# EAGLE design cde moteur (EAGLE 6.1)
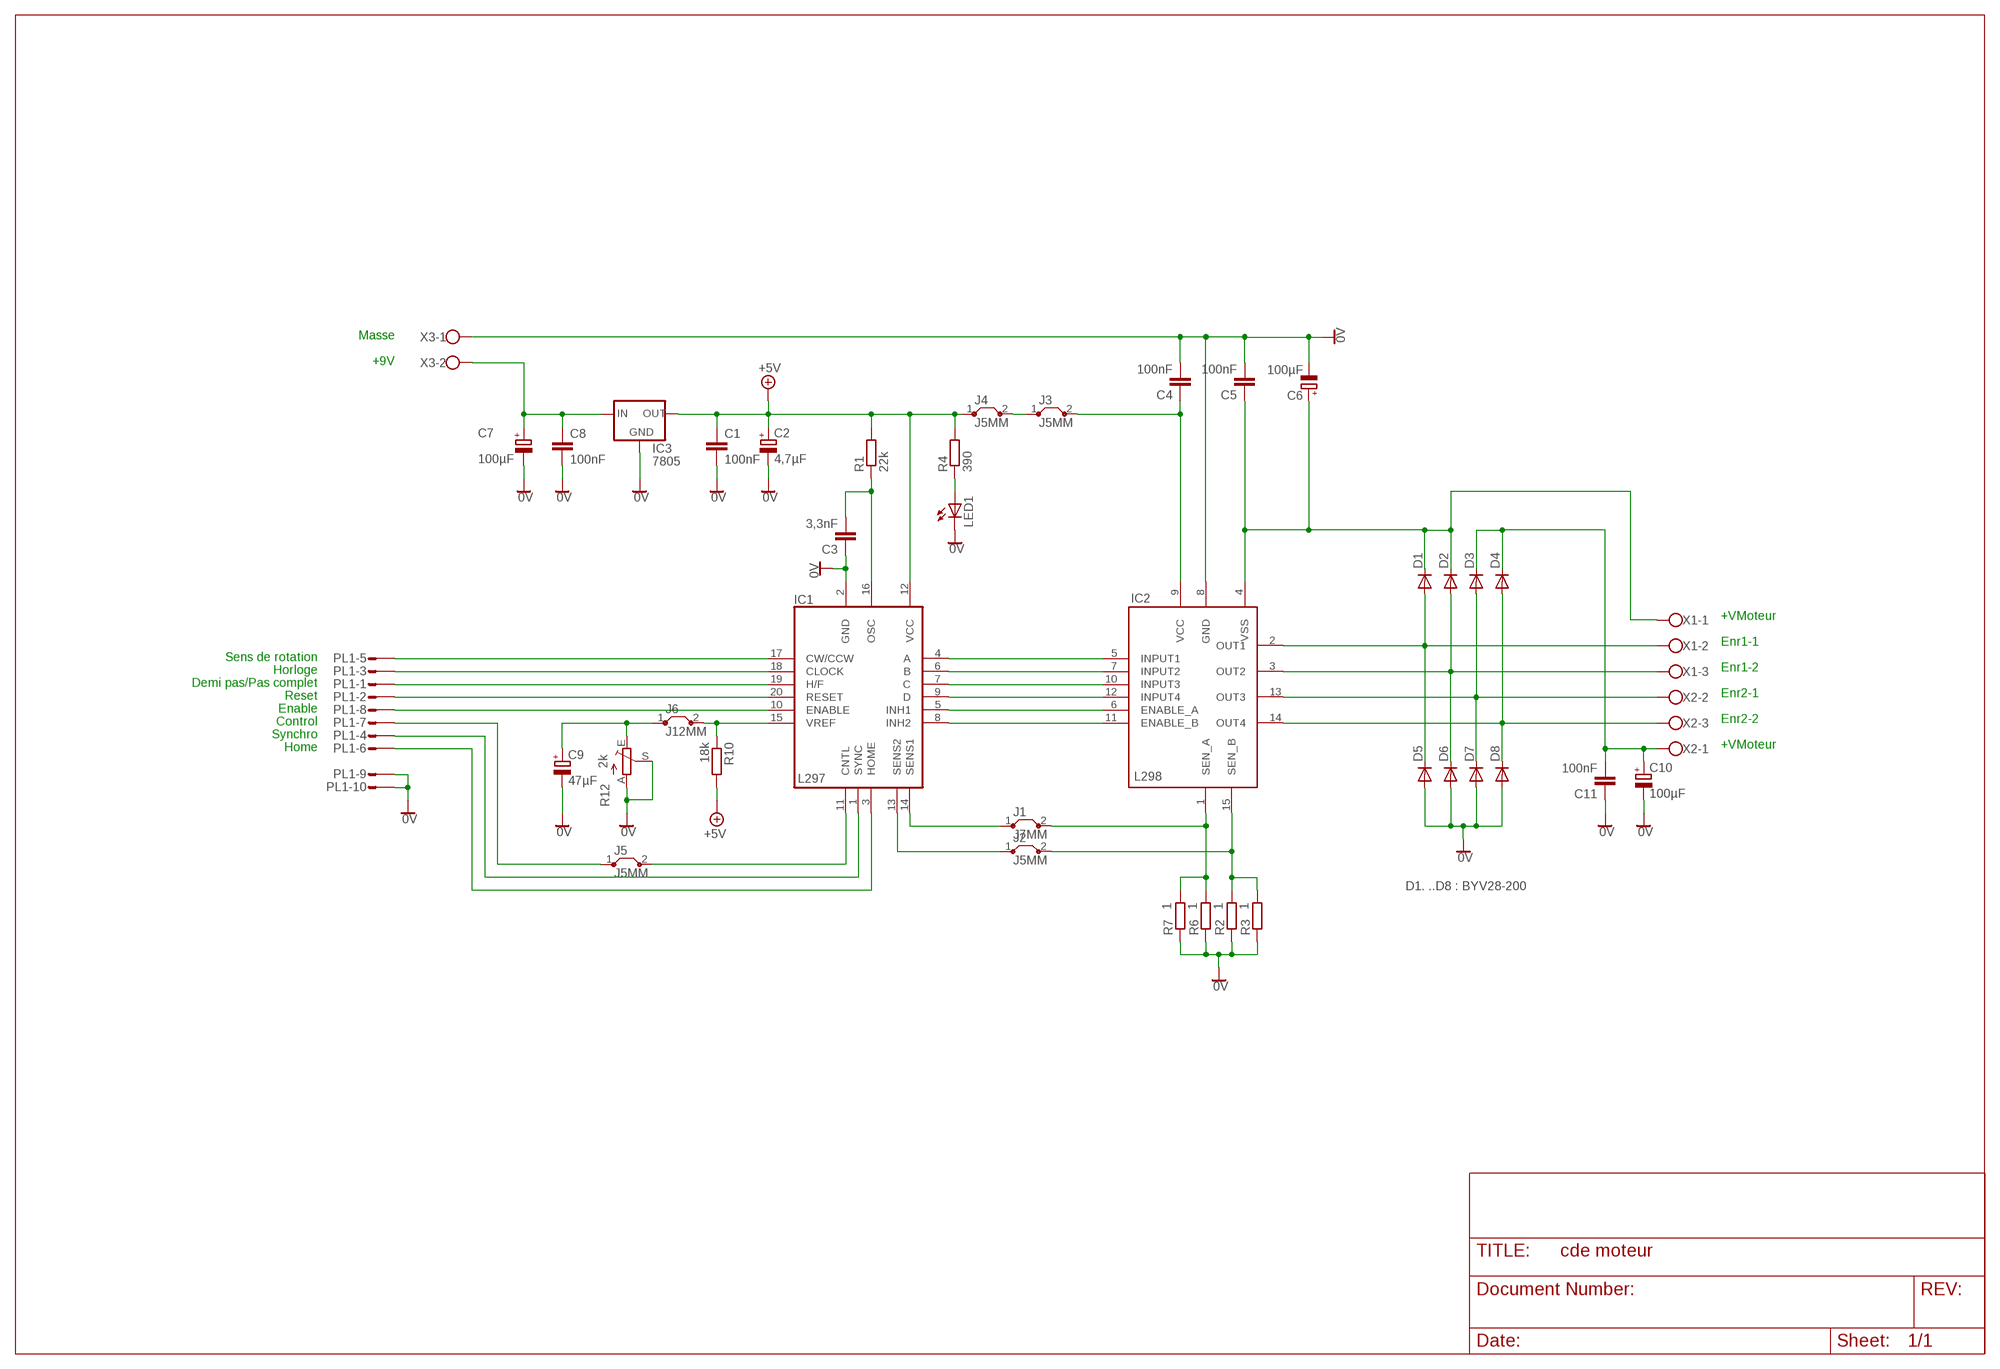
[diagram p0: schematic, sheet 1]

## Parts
C1  100nF  C-EU050-030X075  [C050-030X075]
C2  4,7µF  CPOL-EUE2.5-6  [E2,5-6]
C3  3,3nF  C-EU050-024X044  [C050-024X044]
C4  100nF  C-EU050-030X075  [C050-030X075]
C5  100nF  C-EU050-030X075  [C050-030X075]
C6  100µF  CPOL-EUE5-8.5  [E5-8,5]
C7  100µF  CPOL-EUE2.5-7  [E2,5-7]
C8  100nF  C-EU050-035X075  [C050-035X075]
C9  47µF  CPOL-EUE2.5-6  [E2,5-6]
C10  100µF  CPOL-EUE5-8.5  [E5-8,5]
C11  100nF  C-EU050-030X075  [C050-030X075]
D1  BYW55  [SOD57-10]
D2  BYW55  [SOD57-10]
D3  BYW55  [SOD57-10]
D4  BYW55  [SOD57-10]
D5  BYW55  [SOD57-10]
D6  BYW55  [SOD57-10]
D7  BYW55  [SOD57-10]
D8  BYW55  [SOD57-10]
IC1  L297  [DIL20]
IC2  L298  [MW-15]
IC3  7805  78XXS  [78XXS]
J1  J7MM  [07]
J2  J5MM  [05]
J3  J5MM  [05]
J4  J5MM  [05]
J5  J5MM  [05]
J6  J12MM  [12]
LED1  LED3MM  [LED3MM]
PL1  10HS  [10H]
R1  22k  R-EU_0207/10  [0207/10]
R2  1  R-EU_0309/12  [0309/12]
R3  1  R-EU_0309/12  [0309/12]
R4  390  R-EU_0207/10  [0207/10]
R6  1  R-EU_0309/12  [0309/12]
R7  1  R-EU_0309/12  [0309/12]
R10  18k  R-EU_0207/10  [0207/10]
R12  2k  TRIM_EU-PTSPIN  [PT-SPIN]
X1  W237-103  [W237-103]
X2  W237-103  [W237-103]
X3  W237-102  [W237-102]

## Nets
0V: C1.2 C2.- C3.1 C4.2 C5.2 C6.- C7.- C8.2 C9.- C10.- C11.1 D5.A D6.A D7.A D8.A IC1.2(GND) IC2.8(GND) IC3.GND LED1.K(C) PL1.9 PL1.10 R2.1 R3.1 R6.1 R7.1 R12.A R12.S X3.1
+5V: C1.1 C2.+ IC1.12(VCC) IC3.OUT J4.1 R1.2 R4.2 R10.2
N$1: IC1.4(A) IC2.5(INPUT1)
N$2: IC1.6(B) IC2.7(INPUT2)
N$3: IC1.7(C) IC2.10(INPUT3)
N$4: IC1.9(D) IC2.12(INPUT4)
N$5: IC1.5(INH1) IC2.6(ENABLE_A)
N$6: IC1.8(INH2) IC2.11(ENABLE_B)
N$7: D1.A D5.C IC2.2(OUT1) X1.2
N$8: C3.2 IC1.16(OSC) R1.1
N$9: D2.A D6.C IC2.3(OUT2) X1.3
N$10: D3.A D7.C IC2.13(OUT3) X2.2
N$11: D4.A D8.C IC2.14(OUT4) X2.3
N$12: IC2.1(SEN_A) J1.2 R6.2 R7.2
N$13: C5.1 C6.+ D1.C D2.C IC2.4(VSS) X1.1
N$14: IC2.15(SEN_B) J2.2 R2.2 R3.2
N$15: C7.+ C8.1 IC3.IN X3.2
N$17: C10.+ C11.2 D3.C D4.C X2.1
N$19: IC1.20(RESET) PL1.2
N$20: IC1.19(H/F) PL1.1
N$21: IC1.18(CLOCK) PL1.3
N$22: IC1.17(CW/CCW) PL1.5
N$23: IC1.10(ENABLE) PL1.8
N$24: J5.1 PL1.7
N$25: IC1.1(SYNC) PL1.4
N$26: IC1.3(HOME) PL1.6
N$27: C9.+ J6.1 R12.E
N$29: IC1.14(SENS1) J1.1
N$30: IC1.13(SENS2) J2.1
N$31: C4.1 IC2.9(VCC) J3.2
N$32: J3.1 J4.2
N$33: IC1.11(CNTL) J5.2
N$34: IC1.15(VREF) J6.2 R10.1
N$101: LED1.A R4.1

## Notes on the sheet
- Masse
- +9V
- +VMoteur
- Enr1-1
- Sens de rotation
- Horloge
- Enr1-2
- Demi pas/Pas complet
- Reset
- Enr2-1
- Enable
- Control
- Enr2-2
- Synchro
- Home
- +VMoteur
- D1. ..D8 : BYV28-200

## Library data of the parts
C1 C3-C5 C8 C11 = rcl:C-EU: CAPACITOR, European symbol
C2 C6 C7 C9 C10 = rcl:CPOL-EU: POLARIZED CAPACITOR, European symbol
D1-D8 = diode:BYW55: DIODE
IC1 = sgs-thom:L297
IC2 = sgs-thom:L298
IC3 = v-reg:78XXS: VOLTAGE REGULATOR
J1-J6 = jumper:J: Bridge
LED1 = led:LED: LED
PL1 = con-harting-h:10HS: CONNECTOR
R1-R4 R6 R7 R10 = rcl:R-EU_: RESISTOR, European symbol
R12 = pot:TRIM_EU-: POTENTIOMETER
X1 X2 = con-wago-500:W237-103: WAGO SCREW CLAMP
X3 = con-wago-500:W237-102: WAGO SCREW CLAMP

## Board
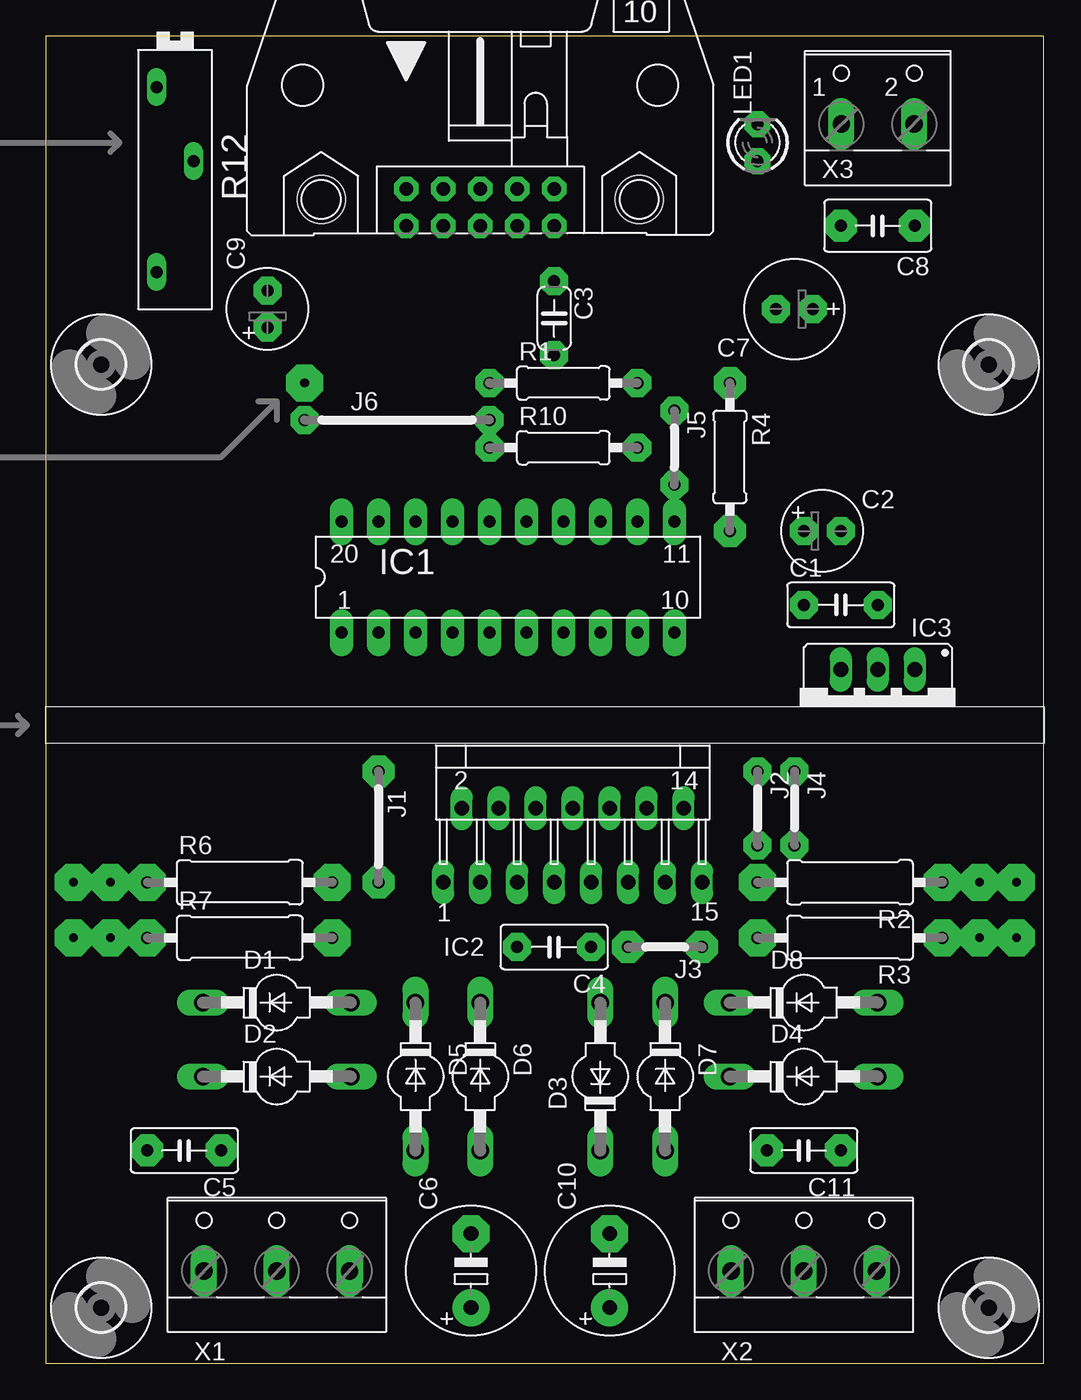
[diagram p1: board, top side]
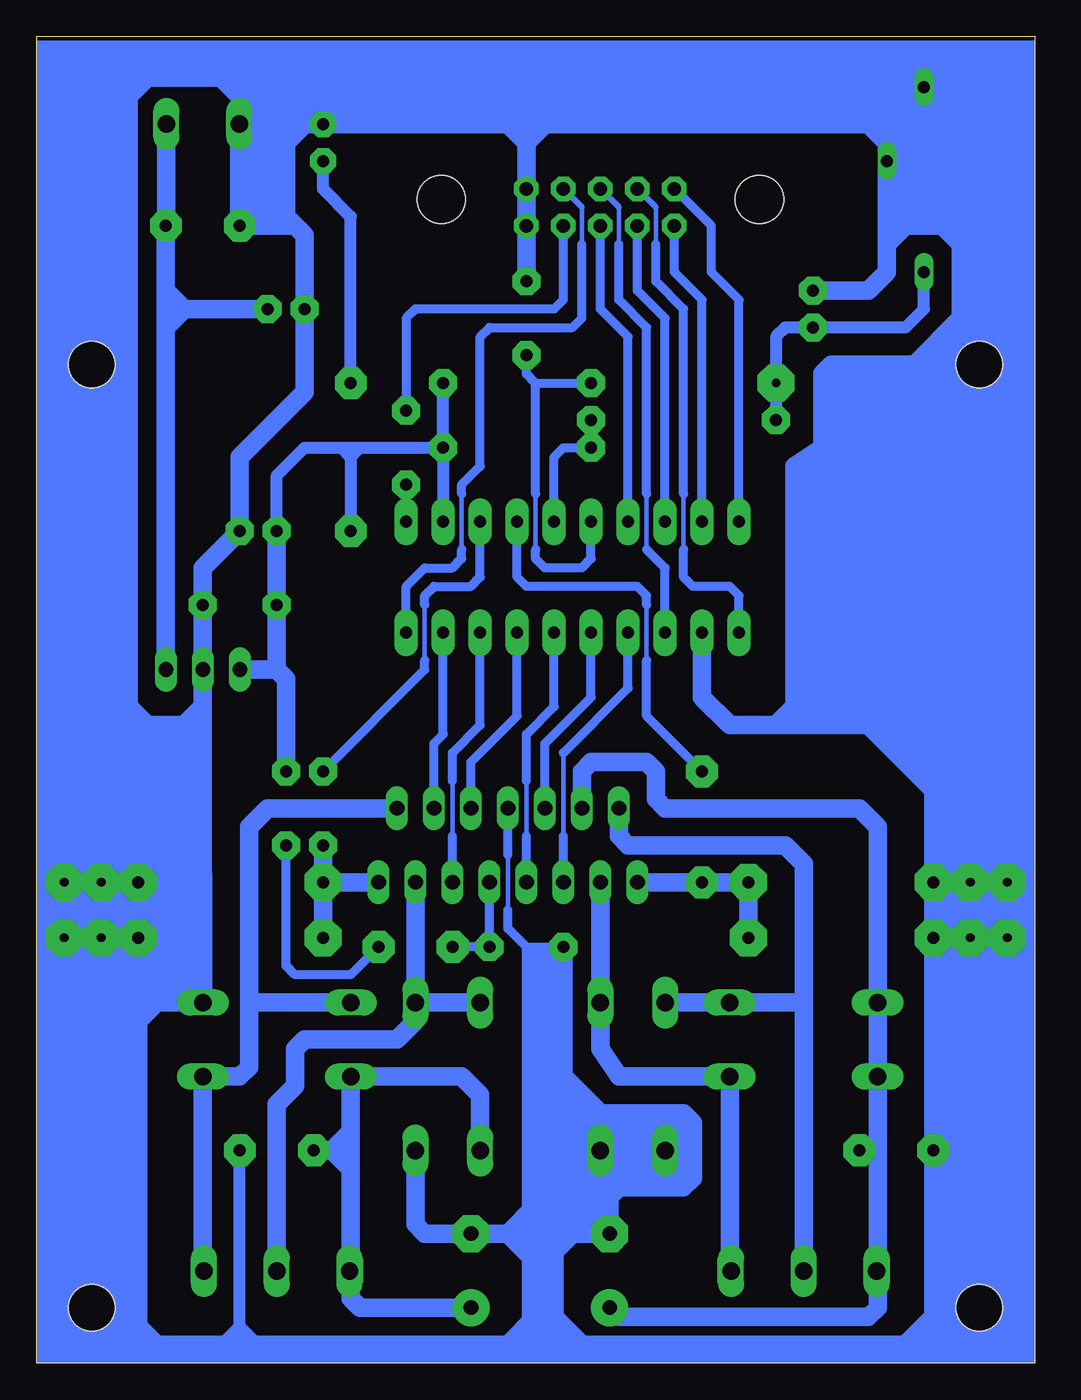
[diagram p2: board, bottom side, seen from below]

Size 68.56 x 91.11 mm. Coordinates in mm from the lower left corner, seen from the top.
Outline: 0,0 68.56,0 68.56,91.11 0,91.11 0,0
Copper layers (1*16): Top 0.035mm / dielectric 1.5mm / Bottom 0.035mm
Design rules: minimum track width 10mil, minimum drill 24mil, track to track 8mil, track to pad 8mil, pad to pad 8mil, via to via 8mil, smd to smd 8mil, copper to edge 40mil, drill to drill 8mil, minimum pad ring 10mil, minimum via ring 8mil, stop-mask expansion 4mil, vias tented up to drill 0mil, thermal gap 10mil

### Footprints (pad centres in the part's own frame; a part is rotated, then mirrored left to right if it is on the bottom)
C050-030X075 = drill 0.813 octagon: 1 -2.54,0; 2 2.54,0
E2,5-6 = drill 0.813 pad 1.6: + -1.27,0 | drill 0.813 pad 1.6 octagon: - 1.27,0
C050-024X044 = drill 0.813 octagon: 1 -2.54,0; 2 2.54,0
E5-8,5 = drill 1.016 pad 2.54: + -2.54,0 | drill 1.016 pad 2.54 octagon: - 2.54,0
E2,5-7 = drill 0.813 pad 1.6: + -1.27,0 | drill 0.813 pad 1.6 octagon: - 1.27,0
C050-035X075 = drill 0.813 octagon: 1 -2.54,0; 2 2.54,0
SOD57-10 = drill 1.194 long: A 5.08,0; C -5.08,0
DIL20 = drill 0.813 pad 1.6 long: 1 -11.43,-3.81; 2 -8.89,-3.81; 3 -6.35,-3.81; 4 -3.81,-3.81; 5 -1.27,-3.81; 6 1.27,-3.81; 7 3.81,-3.81; 8 6.35,-3.81; 9 8.89,-3.81; 10 11.43,-3.81; 11 11.43,3.81; 12 8.89,3.81; 13 6.35,3.81; 14 3.81,3.81; 15 1.27,3.81; 16 -1.27,3.81; 17 -3.81,3.81; 18 -6.35,3.81; 19 -8.89,3.81; 20 -11.43,3.81
MW-15 = drill 1.016 pad 1.27 long: 1 -8.89,-5.08; 2 -7.62,0; 3 -6.35,-5.08; 4 -5.08,0; 5 -3.81,-5.08; 6 -2.54,0; 7 -1.27,-5.08; 8 0,0; 9 1.27,-5.08; 10 2.54,0; 11 3.81,-5.08; 12 5.08,0; 13 6.35,-5.08; 14 7.62,0; 15 8.89,-5.08
78XXS = drill 1.016 long: GND 0,-2.54; IN -2.54,-2.54; OUT 2.54,-2.54
07 = drill 0.813 pad 1.6 octagon: 1 -3.81,0; 2 3.81,0
05 = drill 0.813 pad 1.6 octagon: 1 -2.54,0; 2 2.54,0
12 = drill 0.813 pad 1.6 octagon: 1 -6.35,0; 2 6.35,0
LED3MM = drill 0.813 octagon: A -1.27,0; K 1.27,0
10H = drill 0.914: 1 -5.08,-1.27 | drill 0.914 octagon: 2 -5.08,1.27; 3 -2.54,-1.27; 4 -2.54,1.27; 5 0,-1.27; 6 0,1.27; 7 2.54,-1.27; 8 2.54,1.27; 9 5.08,-1.27; 10 5.08,1.27 | hole 3.302: -10.922,0.533; 10.922,0.533
0207/10 = drill 0.813 octagon: 1 -5.08,0; 2 5.08,0
0309/12 = drill 0.813 octagon: 1 -6.35,0; 2 6.35,0
PT-SPIN = drill 0.813 long: A -6.35,-1.27; E 6.35,-1.27; S -1.27,1.27
3,2 = hole 3.2: 0,0
W237-103 = drill 1.194 long: 1 -5,-1.29; 2 0,-1.29; 3 5,-1.29
W237-102 = drill 1.194 long: 1 -2.5,-1.27; 2 2.5,-1.27

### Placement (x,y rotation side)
C1  54.61,52.07 0 top
C2  53.34,57.15 0 top
C3  34.92,71.76 270 top
C4  34.92,28.57 180 top
C5  9.52,14.61 180 top
C6  29.21,6.35 90 top
C7  51.44,72.39 180 top
C8  57.15,78.11 180 top
C9  15.24,72.39 90 top
C10  38.73,6.35 90 top
C11  52.07,14.61 180 top
D1  15.88,24.77 0 top
D2  15.88,19.68 0 top
D3  38.1,19.68 90 top
D4  52.07,19.68 0 top
D5  25.4,19.68 270 top
D6  29.84,19.68 270 top
D7  42.55,19.68 270 top
D8  52.07,24.77 0 top
IC1  31.75,53.97 0 top
IC2  36.2,38.1 0 top
IC3  57.15,45.08 180 top
J1  22.86,36.83 270 top
J2  48.9,38.1 270 top
J3  42.55,28.57 180 top
J4  51.44,38.1 270 top
J5  43.18,62.87 270 top
J6  24.13,64.77 0 top
LED1  48.9,83.82 90 top
PL1  29.84,79.38 0 top
R1  35.56,67.31 0 top
R2  55.25,33.02 180 top
R3  55.25,29.21 180 top
R4  46.99,62.23 270 top
R6  13.34,33.02 0 top
R7  13.34,29.21 0 top
R10  35.56,62.87 0 top
R12  8.89,81.28 270 top
U$1  [3,2]  3.81,3.81 0 top
U$2  [3,2]  64.77,3.81 0 top
U$3  [3,2]  3.81,68.58 0 top
U$4  [3,2]  64.77,68.58 0 top
X1  15.88,7.62 0 top
X2  52.07,7.62 0 top
X3  57.15,86.36 0 top

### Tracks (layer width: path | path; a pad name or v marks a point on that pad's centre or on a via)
0V
  Bottom 0.305: 36.2,31.11 36.2,34.92
  Bottom 0.406: 10.16,85.09 10.16,85.73 | C8.2 54.65,78.15
  Bottom 0.61: D5.A D6.A 34.92,14.61 | 34.92,28.57 36.2,29.84 36.2,31.11 | 36.2,34.92 IC2.8 | 34.92,14.61 34.92,8.89 34.92,1.27 | 34.92,14.61 34.92,28.57 | 34.92,28.57 C4.2
  Bottom 0.813: 54.61,1.27 54.61,2.54 | 54.61,2.54 C11.1 | 54.61,2.54 55.88,1.27 | 53.34,1.27 54.61,2.54
  Bottom 1.27: 6.98,3.18 6.98,1.9 7.62,1.27 8.89,1.27 | 6.98,3.18 C5.2 6.98,28.57 7.62,29.21 R7.1 R6.1 6.98,39.37 11.43,43.81 16.51,43.81 | 8.89,1.27 31.12,1.27 | 31.12,1.27 34.92,1.27 36.2,1.27 | 36.2,1.27 53.34,1.27 54.61,1.27 55.88,1.27 60.33,1.27 61.59,2.54 61.59,23.5 | 61.59,23.5 61.59,24.77 | 61.59,24.77 61.59,26.04 | 61.59,26.04 R3.1 R2.1 57.79,33.02 57.15,33.65 57.15,45.08 | 61.59,24.77 60.33,24.77 | 60.33,24.77 D8.A | 36.2,8.89 34.92,8.89 31.75,8.89 | 36.2,8.89 C10.- 41.91,8.89 42.55,9.53 D7.A | 31.75,8.89 C6.- | 57.15,45.08 IC3.GND C1.2 57.15,54.61 C2.- 54.61,62.23 50.16,66.67 C7.- 50.16,77.47 50.8,78.11 | 50.8,78.11 51.44,78.11 | 51.44,78.11 C8.2 | 10.16,83.82 R12.S 10.16,78.11 | 10.16,83.82 10.16,85.73 10.16,87 9.52,87.63 R12.A | 11.43,85.09 10.16,85.09 | 33.66,85.09 11.43,85.09 | 34.92,84.45 33.66,85.09 | 34.92,84.45 34.92,83.82 | 34.92,83.82 PL1.10 PL1.9 C3.1 | 16.51,43.81 17.78,43.81 | 17.78,43.81 20.95,43.81 22.86,45.72 IC1.2 | 10.16,76.84 10.16,74.93 11.43,73.66 C9.- | 10.16,78.11 10.16,76.84 | 36.2,85.09 34.92,84.45 | 50.16,85.09 X3.1 54.65,78.15 | 50.16,85.09 LED1.K 36.2,85.09 | 16.51,43.81 16.51,45.08 | 16.51,45.08 16.51,61.59 14.61,62.87 14.61,67.95 13.97,68.58 8.25,68.58 5.08,71.76 5.08,89.54 0.63,89.54 0.63,44.45 | 10.16,78.11 8.89,78.11 | 8.89,78.11 6.35,78.11 | 6.35,78.11 5.71,78.11 4.44,76.84 | 34.92,83.82 33.66,85.09 | 36.2,85.09 34.92,83.82 | 10.16,76.84 8.89,78.11 | 6.35,78.11 4.44,76.2 | 11.43,85.09 10.16,83.82 | 54.61,87 54.61,85.73 | 54.61,87 54.61,87.63 55.25,88.27 55.88,88.27 | 55.88,88.27 60.96,88.27 62.23,87 62.23,45.08 60.96,43.81 58.42,43.81 57.15,45.08 | 61.59,23.5 60.33,24.77 | 60.33,24.77 61.59,26.04
  Bottom 1.27: 36.2,8.89 34.29,10.79 | 36.2,8.89 34.29,6.99 | 36.2,1.27 34.29,3.18 | 33.66,3.18 33.02,3.18 31.12,1.27 | 31.75,8.89 33.02,7.62 | 17.78,43.81 16.51,45.08 | 55.88,88.27 54.61,87 | 6.98,3.18 8.89,1.27 | 51.44,78.11 51.44,83.82 50.16,85.09 | 50.8,78.11 52.07,79.38
+5V
  Bottom 0.813: R10.2 R1.2 | R10.2 IC1.12 | C2.+ 52.07,60.96 50.16,62.87 47.62,62.87 | 47.62,62.87 46.99,62.87 | 46.99,62.87 46.36,62.87 | 46.36,62.87 R10.2 | 46.99,62.87 46.99,62.23 | 46.99,62.23 R4.2 | 46.99,62.23 46.36,62.87 | 46.99,62.23 47.62,62.87
  Bottom 1.27: C2.+ C1.1 52.07,47.62 | 52.07,47.62 IC3.OUT | J4.1 51.44,46.99 52.07,47.62
N$1
  Bottom 0.305: 32.38,36.2 32.38,40 32.38,41.91
  Bottom 0.61: IC1.4 27.94,46.35 32.38,41.91 | IC2.5 32.38,36.2
N$2
  Bottom 0.305: 34.92,36.2 34.92,40
  Bottom 0.61: IC1.6 33.02,45.08 34.92,43.18 34.92,40 | IC2.7 34.92,36.2
N$3
  Bottom 0.61: IC1.7 35.56,44.45 38.73,41.27 IC2.10
N$4
  Bottom 0.61: IC1.9 40.64,43.18 41.27,42.54 IC2.12
N$5
  Bottom 0.61: IC1.5 30.48,45.72 33.66,42.54 IC2.6
N$6
  Bottom 0.305: 40.01,36.2 40.01,40
  Bottom 0.61: IC1.8 38.1,43.81 40.01,41.91 40.01,40 | IC2.11 40.01,36.2
N$7
  Bottom 1.27: D5.C D1.A 15.88,24.77 | X1.2 15.88,24.77 | 15.88,24.77 15.88,34.29 17.14,35.56 27.94,35.56 28.58,36.2 IC2.2
N$8
  Bottom 0.305: 34.29,55.88 34.29,59.69
  Bottom 0.61: 34.29,67.31 R1.1 | 34.29,67.31 34.92,67.95 C3.2 | IC1.16 30.48,55.24 31.12,54.61 33.66,54.61 34.29,55.24 34.29,55.88 | 34.29,59.69 34.29,67.31
N$9
  Bottom 0.406: X1.3 20.95,6.41
  Bottom 1.27: IC2.3 D6.C 29.84,21.59 28.58,19.68 D2.A 20.95,6.41
N$10
  Bottom 1.27: D7.C IC2.13 | D7.C D3.A | D7.C 42.55,23.5 43.82,22.23 50.16,22.23 50.8,21.59 50.8,19.05 52.07,17.78 X2.2
N$11
  Bottom 0.406: X2.3 57.15,6.41
  Bottom 1.27: 53.98,24.77 D8.C | 53.98,24.77 53.98,20.32 54.61,19.68 D4.A 57.15,6.41 | IC2.14 52.7,38.1 53.98,36.83 53.98,24.77
N$12
  Bottom 1.27: R7.2 R6.2 | R6.2 J1.2 | R6.2 IC2.1
N$13
  Bottom 0.406: 10.79,6.41 X1.1 10.79,6.25
  Bottom 0.61: 10.79,14.61 C5.1
  Bottom 1.27: IC2.4 31.12,40.64 30.48,41.27 26.67,41.27 26.03,40.64 26.03,38.73 25.4,38.1 12.06,38.1 10.79,36.83 D1.C D2.C 10.79,14.61 10.79,6.41 | C6.+ 28.58,3.18 11.43,3.18 10.79,3.81 10.79,6.25
N$14
  Bottom 1.27: R2.2 IC2.15 | R3.2 R2.2 | R2.2 J2.2
N$15
  Bottom 0.406: 59.61,78.19 C8.1 59.65,78.15
  Bottom 1.27: 59.69,72.39 59.69,73.66 | 59.69,73.66 C8.1 | 59.69,72.39 58.42,72.39 | 58.42,72.39 C7.+ | 59.65,78.15 X3.2 | IC3.IN 59.69,71.12 | 59.69,71.12 59.69,72.39 | 58.42,72.39 59.69,73.66 | 59.69,71.12 58.42,72.39
N$16  (via drill 0.6 pad 2.54)
  other vias: 4.44,33.02
N$17
  Bottom 0.406: 46.99,6.41 X2.1 46.99,6.25
  Bottom 1.27: D3.C 38.1,18.41 39.37,19.68 D4.C 46.99,15.88 | 46.99,6.41 46.99,13.34 | 46.99,13.34 46.99,14.61 | 46.99,14.61 46.99,15.88 | C10.+ 46.36,3.81 46.99,4.45 46.99,6.25 | 46.99,14.61 48.26,14.61 | 48.26,14.61 C11.2 | 48.26,14.61 46.99,15.88 | 46.99,13.34 48.26,14.61
N$19
  Bottom 0.61: IC1.20 20.32,73.03 22.23,74.93 22.23,78.11 PL1.2
N$20
  Bottom 0.61: IC1.19 22.86,73.03 24.77,74.93 PL1.1
N$21
  Bottom 0.61: IC1.18 25.4,71.76 27.3,73.66 PL1.3
N$22
  Bottom 0.61: IC1.17 27.94,70.48 29.84,72.39 PL1.5
N$23
  Bottom 0.305: 39.37,55.88 39.37,59.69 | 31.12,76.84 31.12,79.38
  Bottom 0.406: 31.12,79.38 PL1.8
  Bottom 0.61: IC1.10 43.18,53.34 41.91,54.61 40.01,54.61 39.37,55.24 39.37,55.88 | 39.37,59.69 39.37,60.32 38.1,61.59 38.1,70.48 37.46,71.12 31.75,71.12 31.12,71.76 31.12,76.84
N$24
  Bottom 0.61: PL1.7 32.38,73.03 33.02,72.39 42.55,72.39 43.18,71.76 J5.1
N$25
  Bottom 0.305: 24.13,55.88 24.13,59.69 | 26.03,76.84 26.03,79.38
  Bottom 0.406: 26.03,79.38 PL1.4
  Bottom 0.61: IC1.1 20.32,52.7 20.95,53.34 23.49,53.34 24.13,53.97 24.13,55.88 | 24.13,59.69 24.13,72.39 26.03,74.3 26.03,76.84
N$26
  Bottom 0.305: 26.67,55.88 26.67,59.69 | 28.58,76.84 28.58,79.38
  Bottom 0.406: 28.58,79.38 PL1.6
  Bottom 0.61: IC1.3 25.4,54.61 26.67,55.88 | 26.67,59.69 26.67,71.12 28.58,73.03 28.58,76.84
N$27  (via drill 0.6 pad 2.54)
  Bottom 0.813: R12.E 7.62,72.39 8.89,71.12 C9.+ 17.14,71.12 17.78,70.48 v17.78,67.31 J6.1
N$29
  Bottom 0.305: 26.67,48.26 26.67,52.07
  Bottom 0.61: J1.1 26.67,44.45 26.67,48.26 | 26.67,52.07 26.67,52.7 27.3,53.34 34.92,53.34 35.56,53.97 IC1.14
N$30
  Bottom 0.305: 41.91,48.26 41.91,52.07
  Bottom 0.61: J2.1 41.91,47.62 41.91,48.26 | 41.91,52.07 41.91,52.7 41.27,53.34 38.73,53.34 38.1,53.97 IC1.13
N$31
  Bottom 0.61: IC2.9 C4.1 J3.2
N$32
  Bottom 0.61: J3.1 46.99,26.67 50.8,26.67 51.44,27.3 J4.2
N$33
  Bottom 0.406: IC1.11 J5.2
N$34
  Bottom 0.61: IC1.15 33.02,62.23 32.38,62.87 R10.1 J6.2
N$35  (via drill 0.6 pad 2.54)
  other vias: 3.81,68.58
N$36  (via drill 0.6 pad 2.54)
  other vias: 64.77,68.58
N$37  (via drill 0.6 pad 2.54)
  other vias: 18.97,79.92
N$38  (via drill 0.6 pad 2.54)
  other vias: 40.78,79.92
N$39  (via drill 0.6 pad 1.68)
  other vias: 24.77,78.11
N$40  (via drill 0.6 pad 1.68)
  other vias: 24.77,80.65
N$41  (via drill 0.6 pad 1.68)
  other vias: 29.84,78.11
N$42  (via drill 0.6 pad 1.68)
  other vias: 27.3,78.11
N$43  (via drill 0.6 pad 1.68)
  other vias: 27.3,80.65
N$44  (via drill 0.6 pad 1.68)
  other vias: 29.84,80.65
N$45  (via drill 0.6 pad 1.68)
  other vias: 32.38,78.11
N$46  (via drill 0.6 pad 1.68)
  other vias: 32.38,80.65
N$47  (via drill 0.6 pad 1.68)
  other vias: 34.92,78.11
N$48  (via drill 0.6 pad 1.68)
  other vias: 34.92,80.65
N$49  (via drill 0.6 pad 2.54)
  other vias: 3.81,3.81
N$50  (via drill 0.6 pad 2.54)
  other vias: 64.77,3.81
N$51  (via drill 0.6 pad 2.18)
  other vias: 49.53,14.61
N$52  (via drill 0.6 pad 2.18)
  other vias: 54.61,14.61
N$53  (via drill 0.6 pad 2.18)
  other vias: 12.06,14.61
N$54  (via drill 0.6 pad 2.18)
  other vias: 6.98,14.61
N$55  (via drill 0.6 pad 2.18)
  other vias: 45.09,28.57
N$56  (via drill 0.6 pad 2.18)
  other vias: 40.01,28.57
N$57  (via drill 0.6 pad 1.93)
  other vias: 37.46,28.57
N$58  (via drill 0.6 pad 1.68, 0.6 pad 1.93)
  Bottom 1.27: v32.38,28.57 32.38,19.68 29.84,17.14 24.13,17.14 23.49,16.51 23.49,12.7 24.13,12.07 28.58,12.07 29.21,11.43 v29.21,8.89
N$59  (via drill 0.6 pad 2.54)
  other vias: 48.9,33.02
N$60  (via drill 0.6 pad 2.54)
  other vias: 61.59,33.02
N$61  (via drill 0.6 pad 2.54)
  other vias: 48.9,29.21
N$62  (via drill 0.6 pad 2.54)
  other vias: 61.59,29.21
N$63  (via drill 0.6 pad 1.93)
  other vias: 48.9,35.56
N$64  (via drill 0.6 pad 1.93)
  other vias: 51.44,35.56
N$65  (via drill 0.6 pad 1.93)
  other vias: 48.9,40.64
N$66  (via drill 0.6 pad 1.93)
  other vias: 51.44,40.64
N$67  (via drill 0.6 pad 1.93)
  other vias: 57.15,52.07
N$68  (via drill 0.6 pad 1.93)
  other vias: 52.07,52.07
N$69  (via drill 0.6 pad 2.18)
  other vias: 22.86,40.64
N$70  (via drill 0.6 pad 2.18)
  other vias: 22.86,33.02
N$71  (via drill 0.6 pad 2.54)
  other vias: 19.69,33.02
N$72  (via drill 0.6 pad 2.54)
  other vias: 19.69,29.21
N$73  (via drill 0.6 pad 2.54)
  other vias: 6.98,33.02
N$74  (via drill 0.6 pad 2.54)
  other vias: 6.98,29.21
N$75  (via drill 0.6 pad 1.93)
  other vias: 30.48,62.87
N$76  (via drill 0.6 pad 1.93)
  other vias: 30.48,64.77
N$77  (via drill 0.6 pad 1.93)
  other vias: 30.48,67.31
N$78  (via drill 0.6 pad 1.93)
  other vias: 17.78,64.77
N$79  (via drill 0.6 pad 1.68)
  other vias: 10.79,6.35
N$80  (via drill 0.6 pad 1.68)
  other vias: 15.88,6.35
N$81  (via drill 0.6 pad 1.68)
  other vias: 20.95,6.35
N$82  (via drill 0.6 pad 1.68)
  other vias: 46.99,6.35
N$83  (via drill 0.6 pad 1.68)
  other vias: 52.07,6.35
N$84  (via drill 0.6 pad 1.68)
  other vias: 57.15,6.35
N$85  (via drill 0.6 pad 1.68)
  other vias: 10.79,19.68
N$86  (via drill 0.6 pad 1.68)
  other vias: 10.79,24.77
N$87  (via drill 0.6 pad 1.68)
  other vias: 20.95,24.77
N$88  (via drill 0.6 pad 1.68)
  other vias: 20.95,19.68
N$89  (via drill 0.6 pad 1.68)
  other vias: 25.4,24.77
N$90  (via drill 0.6 pad 1.68)
  other vias: 29.84,24.77
N$91  (via drill 0.6 pad 1.68)
  other vias: 25.4,14.61
N$92  (via drill 0.6 pad 1.68)
  other vias: 29.84,14.61
N$93  (via drill 0.6 pad 1.68)
  other vias: 46.99,24.77
N$94  (via drill 0.6 pad 1.68)
  other vias: 57.15,24.77
N$95  (via drill 0.6 pad 1.68)
  other vias: 57.15,19.68
N$96  (via drill 0.6 pad 1.68)
  other vias: 46.99,19.68
N$97  (via drill 0.6 pad 1.68)
  other vias: 38.1,24.77
N$98  (via drill 0.6 pad 1.68)
  other vias: 42.55,24.77
N$99  (via drill 0.6 pad 1.68)
  other vias: 42.55,14.61
N$100  (via drill 0.6 pad 1.68)
  other vias: 38.1,14.61
N$101
  Bottom 0.813: R4.1 46.99,78.74 48.9,80.65 LED1.A
N$102  (via drill 0.6 pad 1.68)
  other vias: 29.21,3.81
N$103  (via drill 0.6 pad 1.68)
  other vias: 38.73,3.81
N$104  (via drill 0.6 pad 1.68)
  other vias: 38.73,8.89
N$105  (via drill 0.6 pad 1.27)
  other vias: 28.58,38.1
N$106  (via drill 0.6 pad 1.27)
  other vias: 43.82,38.1
N$107  (via drill 0.6 pad 1.27)
  other vias: 41.27,38.1
N$108  (via drill 0.6 pad 1.27)
  other vias: 38.73,38.1
N$109  (via drill 0.6 pad 1.27)
  other vias: 36.2,38.1
N$110  (via drill 0.6 pad 1.27)
  other vias: 33.66,38.1
N$111  (via drill 0.6 pad 1.27)
  other vias: 31.12,38.1
N$112  (via drill 0.6 pad 1.27)
  other vias: 45.09,33.02
N$113  (via drill 0.6 pad 1.27)
  other vias: 42.55,33.02
N$114  (via drill 0.6 pad 1.27)
  other vias: 40.01,33.02
N$115  (via drill 0.6 pad 1.27)
  other vias: 37.46,33.02
N$116  (via drill 0.6 pad 1.27)
  other vias: 32.38,33.02
N$117  (via drill 0.6 pad 1.27)
  other vias: 34.92,33.02
N$118  (via drill 0.6 pad 1.27)
  other vias: 29.84,33.02
N$119  (via drill 0.6 pad 1.27)
  other vias: 27.3,33.02
N$120  (via drill 0.6 pad 1.27)
  other vias: 54.61,47.62
N$121  (via drill 0.6 pad 1.27)
  other vias: 57.15,47.62
N$122  (via drill 0.6 pad 1.27)
  other vias: 59.69,47.62
N$123  (via drill 0.6 pad 1.27)
  other vias: 20.32,57.78
N$124  (via drill 0.6 pad 1.27)
  other vias: 20.32,50.16
N$125  (via drill 0.6 pad 1.27)
  other vias: 22.86,50.16
N$126  (via drill 0.6 pad 1.27)
  other vias: 25.4,50.16
N$127  (via drill 0.6 pad 1.27)
  other vias: 38.1,57.78
N$128  (via drill 0.6 pad 1.27)
  other vias: 33.02,57.78
N$129  (via drill 0.6 pad 1.27)
  other vias: 27.94,57.78
N$130  (via drill 0.6 pad 1.27)
  other vias: 25.4,57.78
N$131  (via drill 0.6 pad 1.27)
  other vias: 22.86,57.78
N$132  (via drill 0.6 pad 1.27)
  other vias: 30.48,57.78
N$133  (via drill 0.6 pad 1.27)
  other vias: 35.56,57.78
N$134  (via drill 0.6 pad 1.27)
  other vias: 40.64,57.78
N$135  (via drill 0.6 pad 1.27)
  other vias: 43.18,57.78
N$136  (via drill 0.6 pad 1.27)
  other vias: 33.02,50.16
N$137  (via drill 0.6 pad 1.27)
  other vias: 30.48,50.16
N$138  (via drill 0.6 pad 1.27)
  other vias: 27.94,50.16
N$139  (via drill 0.6 pad 1.27)
  other vias: 35.56,50.16
N$140  (via drill 0.6 pad 1.27)
  other vias: 38.1,50.16
N$141  (via drill 0.6 pad 1.27)
  other vias: 40.64,50.16
N$142  (via drill 0.6 pad 1.27)
  other vias: 43.18,50.16
N$143  (via drill 0.6 pad 1.93)
  other vias: 43.18,60.32
N$144  (via drill 0.6 pad 1.93)
  other vias: 43.18,65.41
N$145  (via drill 0.6 pad 1.93)
  other vias: 40.64,62.87
N$146  (via drill 0.6 pad 1.93)
  other vias: 40.64,67.31
N$147  (via drill 0.6 pad 1.93)
  other vias: 34.92,74.3
N$148  (via drill 0.6 pad 1.93)
  other vias: 34.92,69.22
N$149  (via drill 0.6 pad 1.93)
  other vias: 52.7,72.39
N$150  (via drill 0.6 pad 1.93)
  other vias: 50.16,72.39
N$151  (via drill 0.6 pad 1.93)
  other vias: 15.24,73.66
N$152  (via drill 0.6 pad 1.93)
  other vias: 15.24,71.12
N$153  (via drill 0.6 pad 2.18)
  other vias: 54.61,78.11
N$154  (via drill 0.6 pad 2.18)
  other vias: 59.69,78.11
N$155  (via drill 0.6 pad 1.27)
  other vias: 7.62,87.63
N$156  (via drill 0.6 pad 1.27)
  other vias: 10.16,82.55
N$157  (via drill 0.6 pad 1.27)
  other vias: 7.62,74.93
N$158  (via drill 0.6 pad 1.27)
  other vias: 54.61,85.09
N$159  (via drill 0.6 pad 1.27)
  other vias: 59.69,85.09
N$160  (via drill 0.6 pad 1.93)
  other vias: 54.61,57.15
N$161  (via drill 0.6 pad 1.93)
  other vias: 52.07,57.15
N$162  (via drill 0.6 pad 2.18)
  other vias: 46.99,57.15
N$163  (via drill 0.6 pad 2.18)
  other vias: 46.99,67.31
N$164  (via drill 0.6 pad 1.78)
  other vias: 48.9,85.09
N$165  (via drill 0.6 pad 1.78)
  other vias: 48.9,82.55
N$166  (via drill 0.6 pad 2.54)
  other vias: 1.9,33.02
N$167  (via drill 0.6 pad 2.54)
  other vias: 4.44,29.21
N$168  (via drill 0.6 pad 2.54)
  other vias: 1.9,29.21
N$169  (via drill 0.6 pad 2.54)
  other vias: 64.13,33.02
N$170  (via drill 0.6 pad 2.54)
  other vias: 66.67,33.02
N$171  (via drill 0.6 pad 2.54)
  other vias: 66.67,29.21
N$172  (via drill 0.6 pad 2.54)
  other vias: 64.13,29.21
(copper drawn outside any net)
  shapes: Bottom area x51

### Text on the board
tDocu: 0V | +9V | Réglage courant max | Cosse poignard | Prise info courant max | Radiateur constitué | d' une équerre d'alu | A | B | C | D | +24V | +24V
